PROGRAM MAIN_CM
VAR CONSTANT
	cInitFFT	: ST_CM_RealFFT_InitPars := (nFFT_Length := cFFTLength, bHalfSpec := TRUE);														
END_VAR

VAR		
	fbFFT		: FB_CMA_RealFFT := ( stInitPars := cInitFFT, nOwnID := eID_FFT, aDestIDs := [eID_SinkFFT] );										

	(* error monitoring *)
	fbErrHist	: FB_HRErrHist;												
END_VAR

// Call FFT 
fbFFT.Call();
IF fbFFT.bError THEN
	fbErrHist.AddError(bErr:=TRUE, hrErrCode:=fbFFT.hrErrorCode, sErrSource:='MAIN_CM.fbFFT'); // error monitoring
	// ToDo: if error
END_IF

END_PROGRAM
